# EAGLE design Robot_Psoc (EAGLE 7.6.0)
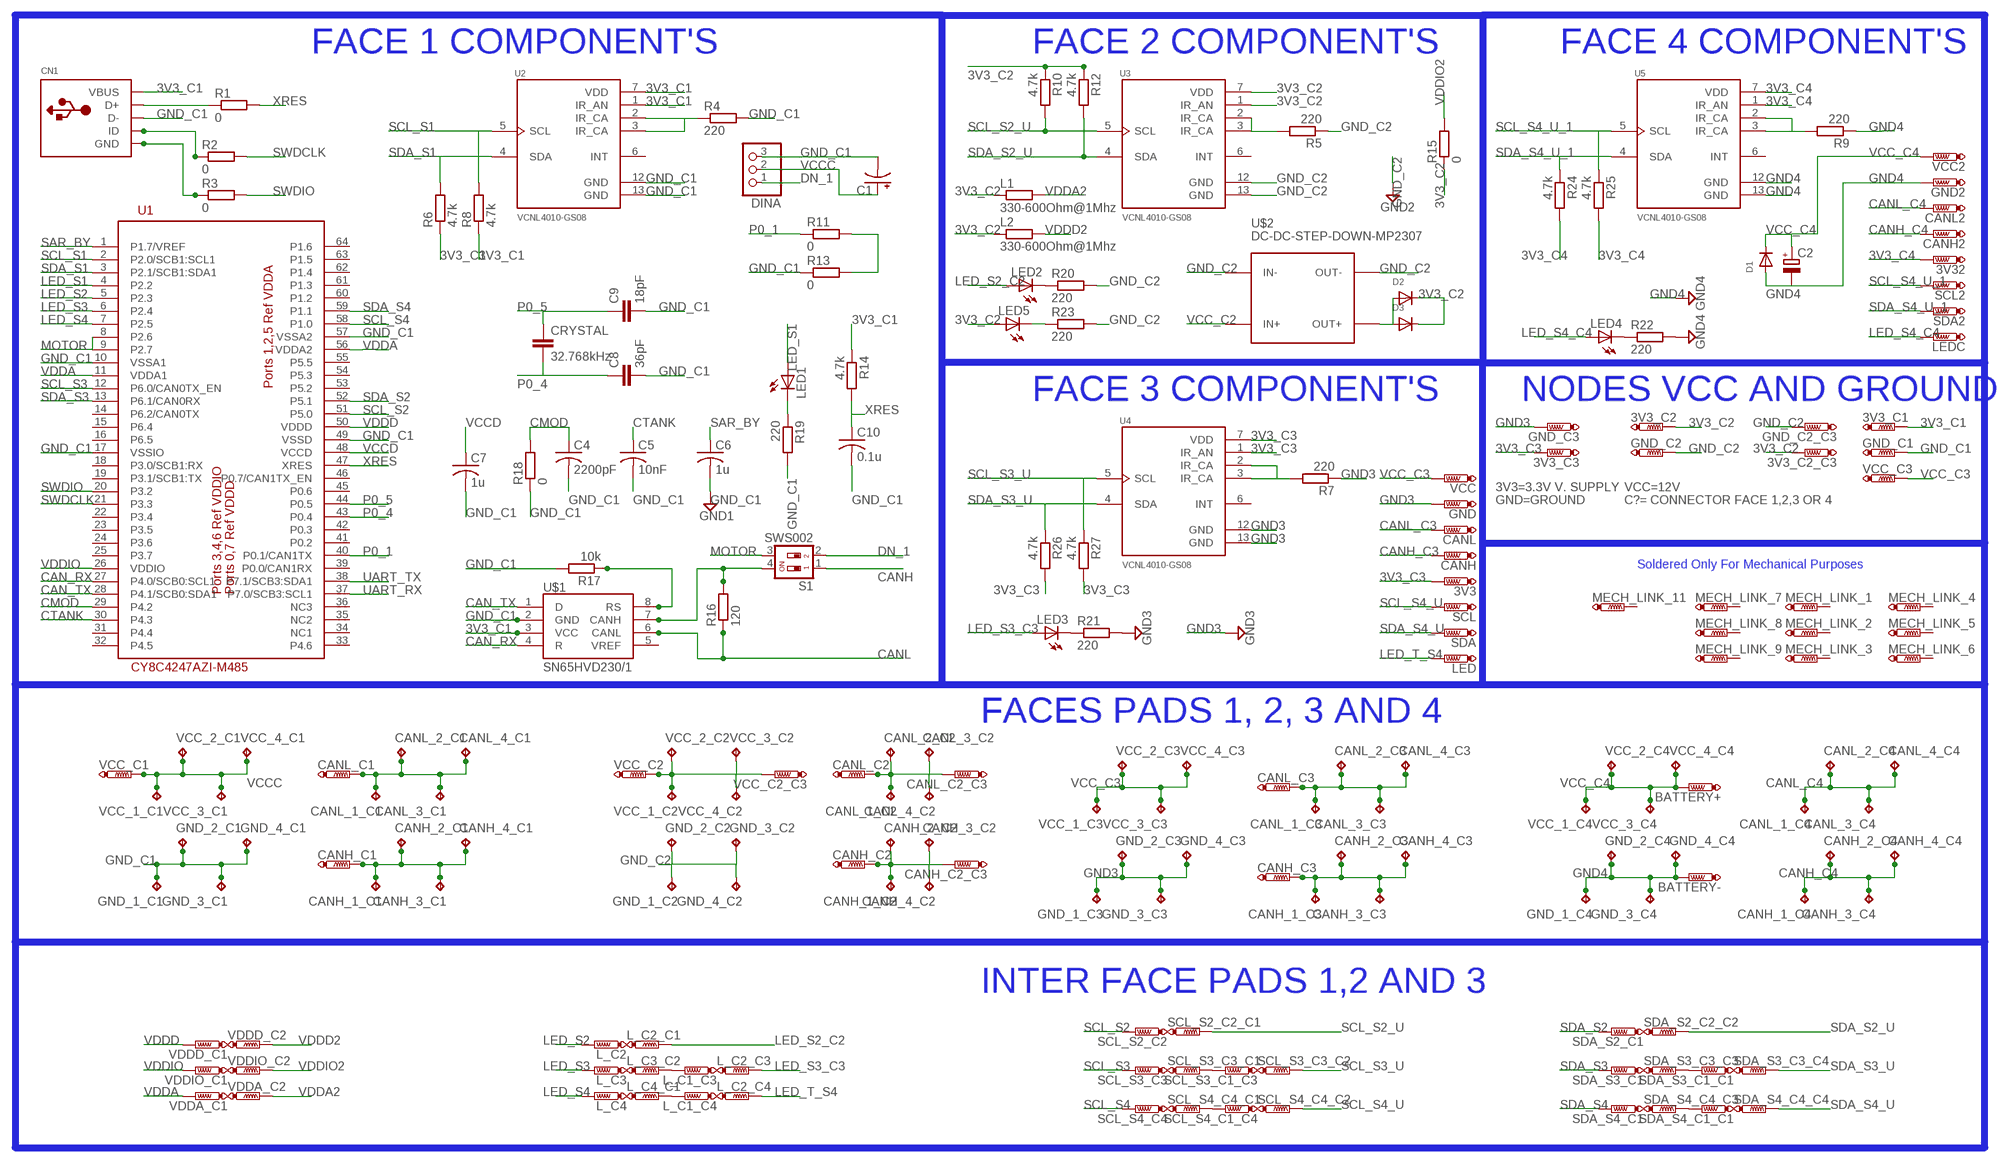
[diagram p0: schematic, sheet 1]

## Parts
3V3  PTR1TP11R  [TP11R]
3V3_C1  PTR1TP11R  [TP11R]
3V3_C2  PTR1TP11R  [TP11R]
3V3_C2_C3  PTR1TP11R  [TP11R]
3V3_C3  PTR1TP11R  [TP11R]
3V32  PTR1TP11R  [TP11R]
BATTERY+  PTR1TP11R  [TP11R]
BATTERY-  PTR1TP11R  [TP11R]
C1  CPOL-USUD-5X5,8  [UD-5X5,8_NICHICON]
C2  CPOL-EUUD-8X10  [UD-8X10_NICHICON]
C4  2200pF  C-USC0805  [C0805]
C5  10nF  C-USC0805  [C0805]
C6  1u  C-USC0805  [C0805]
C7  1u  C-USC0805  [C0805]
C8  36pF  C-EUC0805  [C0805]
C9  18pF  C-EUC0805  [C0805]
C10  0.1u  C-USC0805  [C0805]
CANH  PTR1TP11R  [TP11R]
CANH2  PTR1TP11R  [TP11R]
CANH_1_C1  TPB2,54  [B2,54]
CANH_1_C2  TPB2,54  [B2,54]
CANH_1_C3  TPB2,54  [B2,54]
CANH_1_C4  TPB2,54  [B2,54]
CANH_2_C1  TPB2,54  [B2,54]
CANH_2_C2  TPB2,54  [B2,54]
CANH_2_C3  TPB2,54  [B2,54]
CANH_2_C4  TPB2,54  [B2,54]
CANH_3_C1  TPB2,54  [B2,54]
CANH_3_C2  TPB2,54  [B2,54]
CANH_3_C3  TPB2,54  [B2,54]
CANH_3_C4  TPB2,54  [B2,54]
CANH_4_C1  TPB2,54  [B2,54]
CANH_4_C2  TPB2,54  [B2,54]
CANH_4_C3  TPB2,54  [B2,54]
CANH_4_C4  TPB2,54  [B2,54]
CANH_C1  PTR1TP11R  [TP11R]
CANH_C2  PTR1TP11R  [TP11R]
CANH_C2_C3  PTR1TP11R  [TP11R]
CANH_C3  PTR1TP11R  [TP11R]
CANL  PTR1TP11R  [TP11R]
CANL2  PTR1TP11R  [TP11R]
CANL_1_C1  TPB2,54  [B2,54]
CANL_1_C2  TPB2,54  [B2,54]
CANL_1_C3  TPB2,54  [B2,54]
CANL_1_C4  TPB2,54  [B2,54]
CANL_2_C1  TPB2,54  [B2,54]
CANL_2_C2  TPB2,54  [B2,54]
CANL_2_C3  TPB2,54  [B2,54]
CANL_2_C4  TPB2,54  [B2,54]
CANL_3_C1  TPB2,54  [B2,54]
CANL_3_C2  TPB2,54  [B2,54]
CANL_3_C3  TPB2,54  [B2,54]
CANL_3_C4  TPB2,54  [B2,54]
CANL_4_C1  TPB2,54  [B2,54]
CANL_4_C2  TPB2,54  [B2,54]
CANL_4_C3  TPB2,54  [B2,54]
CANL_4_C4  TPB2,54  [B2,54]
CANL_C1  PTR1TP11R  [TP11R]
CANL_C2  PTR1TP11R  [TP11R]
CANL_C2_C3  PTR1TP11R  [TP11R]
CANL_C3  PTR1TP11R  [TP11R]
CN1  USBMINIB  [USB-MINIB]
CRYSTAL  32.768kHz  C-EUC0603  [C0603]
D1  DIODESMA  [SMADIODE]
D2  DIODESOD-123  [SOD-123]
D3  DIODESOD-123  [SOD-123]
DINA  PINHD-1X3  [1X03]
GND  PTR1TP11R  [TP11R]
GND2  PTR1TP11R  [TP11R]
GND_1_C1  TPB2,54  [B2,54]
GND_1_C2  TPB2,54  [B2,54]
GND_1_C3  TPB2,54  [B2,54]
GND_1_C4  TPB2,54  [B2,54]
GND_2_C1  TPB2,54  [B2,54]
GND_2_C2  TPB2,54  [B2,54]
GND_2_C3  TPB2,54  [B2,54]
GND_2_C4  TPB2,54  [B2,54]
GND_3_C1  TPB2,54  [B2,54]
GND_3_C2  TPB2,54  [B2,54]
GND_3_C3  TPB2,54  [B2,54]
GND_3_C4  TPB2,54  [B2,54]
GND_4_C1  TPB2,54  [B2,54]
GND_4_C2  TPB2,54  [B2,54]
GND_4_C3  TPB2,54  [B2,54]
GND_4_C4  TPB2,54  [B2,54]
GND_C1  PTR1TP11R  [TP11R]
GND_C2  PTR1TP11R  [TP11R]
GND_C2_C3  PTR1TP11R  [TP11R]
GND_C3  PTR1TP11R  [TP11R]
L1  330-600Ohm@1Mhz  R-EU_R0805  [R0805]
L2  330-600Ohm@1Mhz  R-EU_R0805  [R0805]
L_C1_C3  PTR1TP11R  [TP11R]
L_C1_C4  PTR1TP11R  [TP11R]
L_C2  PTR1TP11R  [TP11R]
L_C2_C1  PTR1TP11R  [TP11R]
L_C2_C3  PTR1TP11R  [TP11R]
L_C2_C4  PTR1TP11R  [TP11R]
L_C3  PTR1TP11R  [TP11R]
L_C3_C2  PTR1TP11R  [TP11R]
L_C4  PTR1TP11R  [TP11R]
L_C4_C1  PTR1TP11R  [TP11R]
LED  PTR1TP11R  [TP11R]
LED1  LEDCHIPLED_0805  [CHIPLED_0805]
LED2  LEDCHIPLED_0805  [CHIPLED_0805]
LED3  LEDCHIPLED_0805  [CHIPLED_0805]
LED4  LEDCHIPLED_0805  [CHIPLED_0805]
LED5  LEDCHIPLED_0805  [CHIPLED_0805]
LEDC  PTR1TP11R  [TP11R]
MECH_LINK_1  PTR1TP11R  [TP11R]
MECH_LINK_2  PTR1TP11R  [TP11R]
MECH_LINK_3  PTR1TP11R  [TP11R]
MECH_LINK_4  PTR1TP11R  [TP11R]
MECH_LINK_5  PTR1TP11R  [TP11R]
MECH_LINK_6  PTR1TP11R  [TP11R]
MECH_LINK_7  PTR1TP11R  [TP11R]
MECH_LINK_8  PTR1TP11R  [TP11R]
MECH_LINK_9  PTR1TP11R  [TP11R]
MECH_LINK_11  PTR1TP11R  [TP11R]
R1  0  R-EU_R0805  [R0805]
R2  0  R-EU_R0805  [R0805]
R3  0  R-EU_R0805  [R0805]
R4  220  R-EU_R0805  [R0805]
R5  220  R-EU_R0805  [R0805]
R6  4.7k  R-EU_R0805  [R0805]
R7  220  R-EU_R0805  [R0805]
R8  4.7k  R-EU_R0805  [R0805]
R9  220  R-EU_R0805  [R0805]
R10  4.7k  R-EU_R0805  [R0805]
R11  0  R-EU_R0805  [R0805]
R12  4.7k  R-EU_R0805  [R0805]
R13  0  R-EU_R0805  [R0805]
R14  4.7k  R-EU_R0805  [R0805]
R15  0  R-EU_R0805  [R0805]
R16  120  R-EU_R0805  [R0805]
R17  10k  R-EU_R0805  [R0805]
R18  0  R-EU_R0805  [R0805]
R19  220  R-EU_R0805  [R0805]
R20  220  R-EU_R0805  [R0805]
R21  220  R-EU_R0805  [R0805]
R22  220  R-EU_R0805  [R0805]
R23  220  R-EU_R0805  [R0805]
R24  4.7k  R-EU_R0805  [R0805]
R25  4.7k  R-EU_R0805  [R0805]
R26  4.7k  R-EU_R0805  [R0805]
R27  4.7k  R-EU_R0805  [R0805]
S1  SWS002  [SMS-002]
SCL  PTR1TP11R  [TP11R]
SCL2  PTR1TP11R  [TP11R]
SCL_S2_C2  PTR1TP11R  [TP11R]
SCL_S2_C2_C1  PTR1TP11R  [TP11R]
SCL_S3_C1_C3  PTR1TP11R  [TP11R]
SCL_S3_C3  PTR1TP11R  [TP11R]
SCL_S3_C3_C1  PTR1TP11R  [TP11R]
SCL_S3_C3_C2  PTR1TP11R  [TP11R]
SCL_S4_C1_C4  PTR1TP11R  [TP11R]
SCL_S4_C4  PTR1TP11R  [TP11R]
SCL_S4_C4_C1  PTR1TP11R  [TP11R]
SCL_S4_C4_C2  PTR1TP11R  [TP11R]
SDA  PTR1TP11R  [TP11R]
SDA2  PTR1TP11R  [TP11R]
SDA_S2_C1  PTR1TP11R  [TP11R]
SDA_S2_C2_C2  PTR1TP11R  [TP11R]
SDA_S3_C1  PTR1TP11R  [TP11R]
SDA_S3_C1_C1  PTR1TP11R  [TP11R]
SDA_S3_C3_C3  PTR1TP11R  [TP11R]
SDA_S3_C3_C4  PTR1TP11R  [TP11R]
SDA_S4_C1  PTR1TP11R  [TP11R]
SDA_S4_C1_C1  PTR1TP11R  [TP11R]
SDA_S4_C4_C3  PTR1TP11R  [TP11R]
SDA_S4_C4_C4  PTR1TP11R  [TP11R]
U1  CY8C4247AZI-M485  [TQFP64-10X10]
U2  VCNL4010-GS08  [XDCR_VCNL4010-GS08]
U3  VCNL4010-GS08  [XDCR_VCNL4010-GS08]
U4  VCNL4010-GS08  [XDCR_VCNL4010-GS08]
U5  VCNL4010-GS08  [XDCR_VCNL4010-GS08]
U$1  SN65HVD230/1  [SO8]
U$2  DC-DC-STEP-DOWN-MP2307  [DC-DC-STEP-DOWN-MP2307]
VCC  PTR1TP11R  [TP11R]
VCC2  PTR1TP11R  [TP11R]
VCC_1_C1  TPB2,54  [B2,54]
VCC_1_C2  TPB2,54  [B2,54]
VCC_1_C3  TPB2,54  [B2,54]
VCC_1_C4  TPB2,54  [B2,54]
VCC_2_C1  TPB2,54  [B2,54]
VCC_2_C2  TPB2,54  [B2,54]
VCC_2_C3  TPB2,54  [B2,54]
VCC_2_C4  TPB2,54  [B2,54]
VCC_3_C1  TPB2,54  [B2,54]
VCC_3_C2  TPB2,54  [B2,54]
VCC_3_C3  TPB2,54  [B2,54]
VCC_3_C4  TPB2,54  [B2,54]
VCC_4_C1  TPB2,54  [B2,54]
VCC_4_C2  TPB2,54  [B2,54]
VCC_4_C3  TPB2,54  [B2,54]
VCC_4_C4  TPB2,54  [B2,54]
VCC_C1  PTR1TP11R  [TP11R]
VCC_C2  PTR1TP11R  [TP11R]
VCC_C2_C3  PTR1TP11R  [TP11R]
VCC_C3  PTR1TP11R  [TP11R]
VDDA_C1  PTR1TP11R  [TP11R]
VDDA_C2  PTR1TP11R  [TP11R]
VDDD_C1  PTR1TP11R  [TP11R]
VDDD_C2  PTR1TP11R  [TP11R]
VDDIO_C1  PTR1TP11R  [TP11R]
VDDIO_C2  PTR1TP11R  [TP11R]

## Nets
3V3_C1: 3V3_C1.TP CN1.VBUS R6.1 R8.1 R14.1 U2.1(IR_AN) U2.7(VDD) U$1.3(VCC)
3V3_C2: 3V3_C2.TP 3V3_C2_C3.TP D2.C D3.C L1.1 L2.1 LED5.A R10.1 R12.1 R15.1 U3.1(IR_AN) U3.7(VDD)
3V3_C3: 3V3.TP 3V3_C3.TP R26.2 R27.2 U4.1(IR_AN) U4.7(VDD)
3V3_C4: 3V32.TP R24.2 R25.2 U5.1(IR_AN) U5.7(VDD)
CAN_RX: U1.27(P4.0/SCB0:SCL1) U$1.4(R)
CAN_TX: U1.28(P4.1/SCB0:SDA1) U$1.1(D)
CANH: CANH_1_C1.TP CANH_2_C1.TP CANH_3_C1.TP CANH_4_C1.TP CANH_C1.TP S1.1
CANH_C3: CANH.TP CANH_1_C3.TP CANH_2_C3.TP CANH_3_C3.TP CANH_4_C3.TP CANH_C3.TP
CANH_C4: CANH2.TP CANH_1_C4.TP CANH_2_C4.TP CANH_3_C4.TP CANH_4_C4.TP
CANL: CANL_1_C1.TP CANL_2_C1.TP CANL_3_C1.TP CANL_4_C1.TP CANL_C1.TP R16.1 U$1.6(CANL)
CANL_C3: CANL.TP CANL_1_C3.TP CANL_2_C3.TP CANL_3_C3.TP CANL_4_C3.TP CANL_C3.TP
CANL_C4: CANL2.TP CANL_1_C4.TP CANL_2_C4.TP CANL_3_C4.TP CANL_4_C4.TP
CMOD: C4.1 R18.2 U1.29(P4.2)
CTANK: C5.1 U1.30(P4.3)
DN_1: DINA.1 S1.2
GND3: GND.TP GND_1_C3.TP GND_2_C3.TP GND_3_C3.TP GND_4_C3.TP GND_C3.TP R7.1 R21.2 U4.12(GND) U4.13(GND)
GND4: BATTERY-.TP C2.- D1.A GND2.TP GND_1_C4.TP GND_2_C4.TP GND_3_C4.TP GND_4_C4.TP R9.1 R22.2 U5.12(GND) U5.13(GND)
GND_C1: C1.- C4.2 C5.2 C6.2 C7.2 C8.2 C9.2 C10.2 CN1.D- DINA.3 GND_1_C1.TP GND_2_C1.TP GND_3_C1.TP GND_4_C1.TP GND_C1.TP R4.2 R13.1 R17.2 R18.1 R19.2 U1.10(VSSA1) U1.17(VSSIO) U1.49(VSSD) U1.57(VSSA2) U2.12(GND) U2.13(GND) U$1.2(GND) ; supply symbol labelled GND1
GND_C2: GND_1_C2.TP GND_2_C2.TP GND_3_C2.TP GND_4_C2.TP GND_C2.TP GND_C2_C3.TP R5.1 R20.2 R23.2 U3.12(GND) U3.13(GND) U$2.IN- U$2.OUT- ; supply symbol labelled GND2
LED_S1: LED1.A U1.4(P2.2)
LED_S2: L_C2.TP U1.5(P2.3)
LED_S2_C2: L_C2_C1.TP LED2.A
LED_S3: L_C3.TP U1.6(P2.4)
LED_S3_C3: L_C2_C3.TP LED3.A
LED_S4: L_C4.TP U1.7(P2.5)
LED_S4_C4: LED4.A LEDC.TP
LED_T_S4: L_C2_C4.TP LED.TP
MOTOR: S1.3 U1.8(P2.6) U1.9(P2.7)
N$1: CN1.D+ R1.1
N$2: CN1.ID R2.1
N$3: CN1.GND R3.1
N$4: R11.2 R13.2
N$5: R16.2 S1.4 U$1.7(CANH)
N$7: CANH_1_C2.TP CANH_2_C2.TP CANH_3_C2.TP CANH_4_C2.TP CANH_C2.TP CANH_C2_C3.TP
N$8: R7.2 U4.2(IR_CA) U4.3(IR_CA)
N$9: R17.1 U$1.8(RS)
N$10: SDA_S3_C1_C1.TP SDA_S3_C3_C3.TP
N$14: LED1.C R19.1
N$15: LED2.C R20.1
N$16: LED3.C R21.1
N$17: LED4.C R22.1
N$18: LED5.C R23.1
N$20: L_C1_C4.TP L_C4_C1.TP
N$21: R4.1 U2.2(IR_CA) U2.3(IR_CA)
N$22: L_C1_C3.TP L_C3_C2.TP
N$24: D2.A D3.A U$2.OUT+
N$26: SCL_S3_C1_C3.TP SCL_S3_C3_C1.TP
N$27: SCL_S4_C1_C4.TP SCL_S4_C4_C1.TP
N$32: CANL_1_C2.TP CANL_2_C2.TP CANL_3_C2.TP CANL_4_C2.TP CANL_C2.TP CANL_C2_C3.TP
N$43: R5.2 U3.2(IR_CA) U3.3(IR_CA)
N$44: SDA_S4_C1_C1.TP SDA_S4_C4_C3.TP
N$46: R9.2 U5.2(IR_CA) U5.3(IR_CA)
P0_1: R11.1 U1.40(P0.1/CAN1TX)
P0_4: C8.1 CRYSTAL.2 U1.43(P0.4)
P0_5: C9.1 CRYSTAL.1 U1.44(P0.5)
SAR_BY: C6.1 U1.1(P1.7/VREF)
SCL_S1: R8.2 U1.2(P2.0/SCB1:SCL1) U2.5(SCL)
SCL_S2: SCL_S2_C2.TP U1.51(P5.0)
SCL_S2_U: R10.2 SCL_S2_C2_C1.TP U3.5(SCL)
SCL_S3: SCL_S3_C3.TP U1.12(P6.0/CAN0TX_EN)
SCL_S3_U: R27.1 SCL_S3_C3_C2.TP U4.5(SCL)
SCL_S4: SCL_S4_C4.TP U1.58(P1.0)
SCL_S4_U: SCL.TP SCL_S4_C4_C2.TP
SCL_S4_U_1: R25.1 SCL2.TP U5.5(SCL)
SDA_S1: R6.2 U1.3(P2.1/SCB1:SDA1) U2.4(SDA)
SDA_S2: SDA_S2_C1.TP U1.52(P5.1)
SDA_S2_U: R12.2 SDA_S2_C2_C2.TP U3.4(SDA)
SDA_S3: SDA_S3_C1.TP U1.13(P6.1/CAN0RX)
SDA_S3_U: R26.1 SDA_S3_C3_C4.TP U4.4(SDA)
SDA_S4: SDA_S4_C1.TP U1.59(P1.1)
SDA_S4_U: SDA.TP SDA_S4_C4_C4.TP
SDA_S4_U_1: R24.1 SDA2.TP U5.4(SDA)
SWDCLK: R2.2 U1.21(P3.3)
SWDIO: R3.2 U1.20(P3.2)
UART_RX: U1.37(P7.0/SCB3:SCL1)
UART_TX: U1.38(P7.1/SCB3:SDA1)
VCC_C2: U$2.IN+ VCC_1_C2.TP VCC_2_C2.TP VCC_3_C2.TP VCC_4_C2.TP VCC_C2.TP VCC_C2_C3.TP
VCC_C3: VCC.TP VCC_1_C3.TP VCC_2_C3.TP VCC_3_C3.TP VCC_4_C3.TP VCC_C3.TP
VCC_C4: BATTERY+.TP C2.+ D1.C VCC2.TP VCC_1_C4.TP VCC_2_C4.TP VCC_3_C4.TP VCC_4_C4.TP
VCCC: C1.+ DINA.2 VCC_1_C1.TP VCC_2_C1.TP VCC_3_C1.TP VCC_4_C1.TP VCC_C1.TP
VCCD: C7.1 U1.48(VCCD)
VDDA: U1.11(VDDA1) U1.56(VDDA2) VDDA_C1.TP
VDDA2: L1.2 VDDA_C2.TP
VDDD: U1.50(VDDD) VDDD_C1.TP
VDDD2: L2.2 VDDD_C2.TP
VDDIO: U1.26(VDDIO) VDDIO_C1.TP
VDDIO2: R15.2 VDDIO_C2.TP
XRES: C10.1 R1.2 R14.2 U1.47(XRES)
Unconnected: MECH_LINK_1.TP MECH_LINK_2.TP MECH_LINK_3.TP MECH_LINK_4.TP MECH_LINK_5.TP MECH_LINK_6.TP MECH_LINK_7.TP MECH_LINK_8.TP MECH_LINK_9.TP MECH_LINK_11.TP U1.14(P6.2/CAN0TX) U1.15(P6.4) U1.16(P6.5) U1.18(P3.0/SCB1:RX) U1.19(P3.1/SCB1:TX) U1.22(P3.4) U1.23(P3.5) U1.24(P3.6) U1.25(P3.7) U1.31(P4.4) U1.32(P4.5) U1.33(P4.6) U1.34(NC1) U1.35(NC2) U1.36(NC3) U1.39(P0.0/CAN1RX) U1.41(P0.2) U1.42(P0.3) U1.45(P0.6) U1.46(P0.7/CAN1TX_EN) U1.53(P5.2) U1.54(P5.3) U1.55(P5.5) U1.60(P1.2) U1.61(P1.3) U1.62(P1.4) U1.63(P1.5) U1.64(P1.6) U2.6(INT) U3.6(INT) U4.6(INT) U5.6(INT) U$1.5(VREF)

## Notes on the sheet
- FACE 1 COMPONENT'S | FACE 2 COMPONENT'S | FACE 4 COMPONENT'S
- FACE 3 COMPONENT'S | NODES VCC AND GROUND
- 3V3=3.3V V. SUPPLY | VCC=12V
- GND=GROUND | C?= CONNECTOR FACE 1,2,3 OR 4
- Soldered Only For Mechanical Purposes
- FACES PADS 1, 2, 3 AND 4
- INTER FACE PADS 1,2 AND 3

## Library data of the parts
3V3 3V3_C1 3V3_C2 3V3_C2_C3 3V3_C3 3V32 BATTERY+ BATTERY- CANH CANH2 CANH_C1 CANH_C2 CANH_C2_C3 CANH_C3 CANL CANL2 CANL_C1 CANL_C2 CANL_C2_C3 CANL_C3 GND GND2 GND_C1 GND_C2 GND_C2_C3 GND_C3 L_C1_C3 L_C1_C4 L_C2 L_C2_C1 L_C2_C3 L_C2_C4 L_C3 L_C3_C2 L_C4 L_C4_C1 LED LEDC MECH_LINK_1-MECH_LINK_9 MECH_LINK_11 SCL SCL2 SCL_S2_C2 SCL_S2_C2_C1 SCL_S3_C1_C3 SCL_S3_C3 SCL_S3_C3_C1 SCL_S3_C3_C2 SCL_S4_C1_C4 SCL_S4_C4 SCL_S4_C4_C1 SCL_S4_C4_C2 SDA SDA2 SDA_S2_C1 SDA_S2_C2_C2 SDA_S3_C1 SDA_S3_C1_C1 SDA_S3_C3_C3 SDA_S3_C3_C4 SDA_S4_C1 SDA_S4_C1_C1 SDA_S4_C4_C3 SDA_S4_C4_C4 VCC VCC2 VCC_C1 VCC_C2 VCC_C2_C3 VCC_C3 VDDA_C1 VDDA_C2 VDDD_C1 VDDD_C2 VDDIO_C1 VDDIO_C2 = testpad:PTR1: TEST PIN
C1 = rcl:CPOL-US: POLARIZED CAPACITOR, American symbol
C2 = rcl:CPOL-EU: POLARIZED CAPACITOR, European symbol
C4-C7 C10 = rcl:C-US: CAPACITOR, American symbol
C8 C9 CRYSTAL = rcl:C-EU: CAPACITOR, European symbol
CANH_1_C1-CANH_1_C4 CANH_2_C1-CANH_2_C4 CANH_3_C1-CANH_3_C4 CANH_4_C1-CANH_4_C4 CANL_1_C1-CANL_1_C4 CANL_2_C1-CANL_2_C4 CANL_3_C1-CANL_3_C4 CANL_4_C1-CANL_4_C4 GND_1_C1-GND_1_C4 GND_2_C1-GND_2_C4 GND_3_C1-GND_3_C4 GND_4_C1-GND_4_C4 VCC_1_C1-VCC_1_C4 VCC_2_C1-VCC_2_C4 VCC_3_C1-VCC_3_C4 VCC_4_C1-VCC_4_C4 = testpad:TP: Test pad
CN1 = adafruit:USB: USB Connectors USBMINIB - Surface Mount Female Mini-B USB Connector 4UConnector: 06564 By microbuilder.eu Thru-hole RA Female Mini-B USB Connector 4UConnector: 18732 By ladyada.net
D1-D3 = adafruit:DIODE: Diode
DINA = pinhead:PINHD-1X3: PIN HEADER
L1 L2 R1-R27 = rcl:R-EU_: RESISTOR, European symbol
LED1-LED5 = adafruit:LED: LED
S1 = smd-special:SWS002: SMD Dip Switch 2 pol.
U1 = CypressPSoC:CY8C4247AZI-M485
U2-U5 = VCNL4010-GS08:VCNL4010-GS08
U$1 = texas_instruments:SN65HVD230/1
U$2 = diy-modules:DC-DC-STEP-DOWN-MP2307: DC/DC Step-Down Regulator based on MP2307DN chip MP2307 datasheet available here: https://cdn-shop.adafruit.com/datasheets/MP2307_r1.9.pdf Click here to find device on ebay.com

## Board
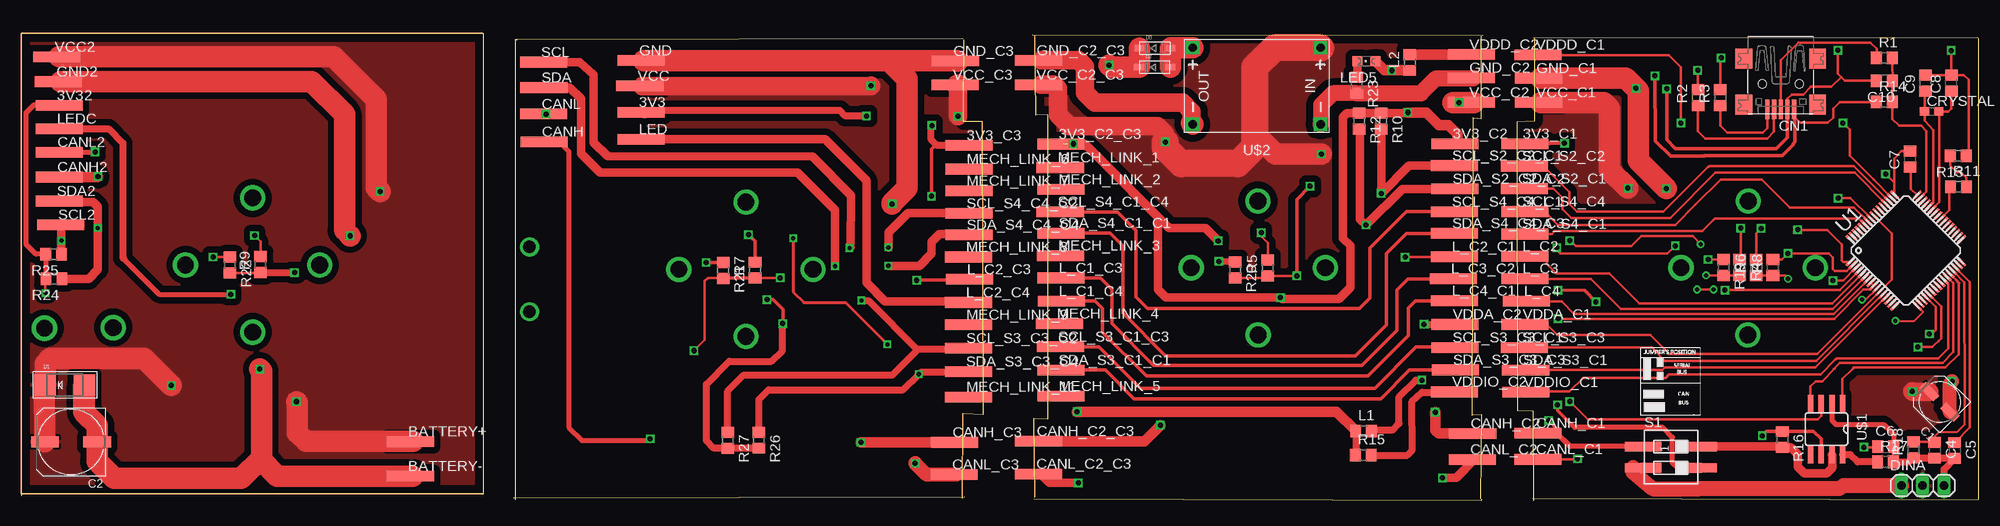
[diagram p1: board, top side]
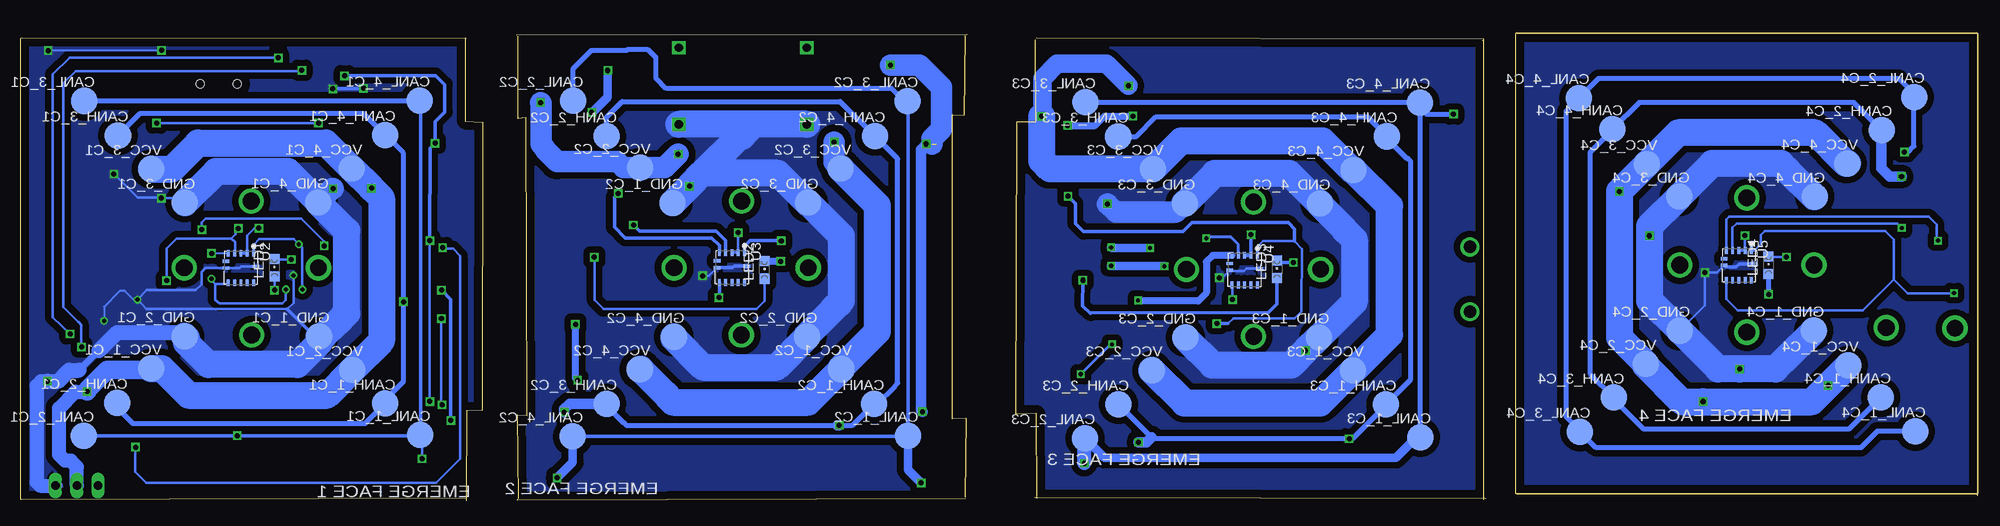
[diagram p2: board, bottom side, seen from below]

Size 233.48 x 55.82 mm. Coordinates in mm from the lower left corner, seen from the top.
Outline: 120.64,55.61 174.37,55.53
Outline: 112.44,55.01 112.4,45.25 114.65,45.24 114.75,10.31 112.3,10.39 112.28,0.29
Outline: 174.09,0.24 174.22,10.24 173.12,10.2 173.22,45.7 174.14,45.57 174.14,55.44
Outline: 120.84,55.49 120.94,46.04 122.4,46.1 122.4,9.76 120.75,9.84 120.86,0.38
Outline: 180.37,0 180.3,10.7 178.47,10.75 178.42,45.2 180.47,45.3 180.47,55.29
Outline: 0.01,0.55 0.01,55.55
Outline: 112.49,0.41 58.72,0.29
Outline: 112.33,55.19 58.97,55.08 58.97,0.08
Outline: 0,0.78 0,55.78
Outline: 233.37,55.26 180.34,55.2
Outline: 180.34,0.3 233.43,0.1
Outline: 233.48,0.17 233.48,55.17
Outline: 120.76,0.25 174.21,0.06 174.24,0.13
Outline: 59.12,54.99 59.01,54.99
Outline: 0.12,0.82 55.12,0.82 55.12,55.82 0.12,55.82
Outline: 55.01,0.82 0.01,0.82 0.01,55.82 55.01,55.82
Copper layers (1*16): Top 0.035mm / dielectric 1.5mm / Bottom 0.035mm
Design rules "default": minimum track width 10mil, minimum drill 24mil, track to track 8mil, track to pad 8mil, pad to pad 8mil, via to via 8mil, smd to smd 8mil, copper to edge 40mil, drill to drill 8mil, minimum pad ring 10mil, minimum via ring 8mil, stop-mask expansion 4mil, vias tented up to drill 0mil, thermal gap 10mil

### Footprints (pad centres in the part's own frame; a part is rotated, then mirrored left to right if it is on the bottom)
TP11R = smd 0.635 x 1.27: P$1 0.381,0; P$2 1.016,0; P$3 -0.254,0; P$4 -0.889,0; P$5 -1.524,0; P$6 1.613,0; P$7 2.21,0; P$8 -2.146,0; P$9 -2.769,0 | smd 1.1 x 1.1: TP 0,0
UD-5X5,8_NICHICON = smd 2.3 x 1: + 1.725,0; - -1.7,0
UD-8X10_NICHICON = smd 3.3 x 1.3: + 3.125,0; - -3.125,0
C0805 = smd 1.3 x 1.5: 1 -0.95,0; 2 0.95,0
B2,54 = smd 3.175 x 3.175 bottom: P$1 0,0 | smd 2.54 x 2.54 bottom: TP 0,0
USB-MINIB = smd 0.5 x 2.308: D+ 0,4.064; D- -0.8,4.064; GND 1.6,4.064; ID 0.8,4.064; VBUS -1.6,4.064 | smd 2 x 2.4: GND1 -4.4,-2; GND2 -4.4,3.5; GND3 4.4,3.5; GND4 4.4,-2 | hole 1: -2.2,1; 2.2,1
C0603 = smd 1.1 x 1: 1 -0.85,0; 2 0.85,0
SMADIODE = smd 2.54 x 2.54: A 2.349,0; C -2.349,0
SOD-123 = smd 1.2 x 0.7: A 1.85,0; C -1.85,0
1X03 = drill 1.016 long: 1 -2.54,0; 2 0,0; 3 2.54,0
R0805 = smd 1.3 x 1.5: 1 -0.95,0; 2 0.95,0
CHIPLED_0805 = smd 1.2 x 1.2: A 0,-1.05; C 0,1.05
SMS-002 = smd 1.092 x 2.007: 1 -1.27,-4.496; 2 1.27,-4.496; 3 1.27,4.496; 4 -1.27,4.496 | smd 1.143 x 2.54: P$1 -1.27,2.413; P$2 1.27,2.413; P$3 -1.27,-2.413; P$4 1.27,-2.413
TQFP64-10X10 = smd 1.2 x 0.3: 1 -5.7,3.75; 2 -5.7,3.25; 3 -5.7,2.75; 4 -5.7,2.25; 5 -5.7,1.75; 6 -5.7,1.25; 7 -5.7,0.75; 8 -5.7,0.25; 9 -5.7,-0.25; 10 -5.7,-0.75; 11 -5.7,-1.25; 12 -5.7,-1.75; 13 -5.7,-2.25; 14 -5.7,-2.75; 15 -5.7,-3.25; 16 -5.7,-3.75; 33 5.7,-3.75; 34 5.7,-3.25; 35 5.7,-2.75; 36 5.7,-2.25; 37 5.7,-1.75; 38 5.7,-1.25; 39 5.7,-0.75; 40 5.7,-0.25; 41 5.7,0.25; 42 5.7,0.75; 43 5.7,1.25; 44 5.7,1.75; 45 5.7,2.25; 46 5.7,2.75; 47 5.7,3.25; 48 5.7,3.75 | smd 0.3 x 1.2: 17 -3.75,-5.7; 18 -3.25,-5.7; 19 -2.75,-5.7; 20 -2.25,-5.7; 21 -1.75,-5.7; 22 -1.25,-5.7; 23 -0.75,-5.7; 24 -0.25,-5.7; 25 0.25,-5.7; 26 0.75,-5.7; 27 1.25,-5.7; 28 1.75,-5.7; 29 2.25,-5.7; 30 2.75,-5.7; 31 3.25,-5.7; 32 3.75,-5.7; 49 3.75,5.7; 50 3.25,5.7; 51 2.75,5.7; 52 2.25,5.7; 53 1.75,5.7; 54 1.25,5.7; 55 0.75,5.7; 56 0.25,5.7; 57 -0.25,5.7; 58 -0.75,5.7; 59 -1.25,5.7; 60 -1.75,5.7; 61 -2.25,5.7; 62 -2.75,5.7; 63 -3.25,5.7; 64 -3.75,5.7
XDCR_VCNL4010-GS08 = smd 0.805 x 0.35: 1 -1.772,1.5; 2 -1.772,0.75; 3 -1.772,0; 4 -1.772,-0.75; 5 -1.772,-1.5; 7 1.772,-1.5; 8 1.772,-0.75; 9 1.772,0; 10 1.772,0.75; 11 1.772,1.5 | smd 0.4 x 0.805: 6 -0.8,-1.772; 12 -0.175,1.772; 13 0,-1.772
SO8 = smd 0.66 x 2.032: 1 -1.905,-3.073; 2 -0.635,-3.073; 3 0.635,-3.073; 4 1.905,-3.073; 5 1.905,3.073; 6 0.635,3.073; 7 -0.635,3.073; 8 -1.905,3.073
DC-DC-STEP-DOWN-MP2307 = drill 1 pad 1.6 square: IN+ -7.62,-4.572; IN- -7.62,4.572; OUT+ 7.62,-4.572; OUT- 7.62,4.572

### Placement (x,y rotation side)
3V3  74.2,46.36 0 top
3V3_C1  179.65,42.6 0 top
3V3_C2  171.29,42.6 0 top
3V3_C2_C3  124.28,42.55 0 top
3V3_C3  113.3,42.39 0 top
3V32  4.77,47.17 0 top
BATTERY+  46.7,7.05 0 top
BATTERY-  46.68,2.91 0 top
C1  228.85,11.76 135 top
C2  5.91,7 180 top
C4  228.24,6.02 270 top
C5  230.63,5.97 270 top
C6  222.4,6.43 0 top
C7  225.32,40.77 90 top
C8  230.25,49.84 90 top
C9  227.17,49.84 90 top
C10  222.22,50.12 180 top
CANH  62.61,42.84 0 top
CANH2  4.79,38.61 0 top
CANH_1_C1  190.04,11.58 0 top
CANH_1_C2  131.73,11.53 0 top
CANH_1_C3  70.64,11.47 0 top
CANH_1_C4  11.62,12.33 0 top
CANH_2_C1  222,11.67 0 top
CANH_2_C2  163.62,43.48 0 top
CANH_2_C3  102.52,11.47 0 top
CANH_2_C4  11.48,44.25 0 top
CANH_3_C1  221.9,43.59 0 top
CANH_3_C2  163.62,11.55 0 top
CANH_3_C3  102.58,43.46 0 top
CANH_3_C4  43.44,12.3 0 top
CANH_4_C1  190.01,43.65 0 top
CANH_4_C2  131.6,43.52 0 top
CANH_4_C3  70.51,43.48 0 top
CANH_4_C4  43.61,44.33 0 top
CANH_C1  181.2,8.06 0 top
CANH_C2  173.4,8 0 top
CANH_C2_C3  121.64,7.09 0 top
CANH_C3  111.59,6.95 0 top
CANL  62.57,46.14 0 top
CANL2  4.8,41.59 0 top
CANL_1_C1  185.87,7.83 0 top
CANL_1_C2  127.66,7.73 0 top
CANL_1_C3  66.5,7.56 0 top
CANL_1_C4  7.48,8.27 0 top
CANL_2_C1  225.99,7.74 0 top
CANL_2_C2  167.63,47.73 0 top
CANL_2_C3  106.56,7.45 0 top
CANL_2_C4  7.6,48.19 0 top
CANL_3_C1  225.91,47.72 0 top
CANL_3_C2  127.68,47.68 0 top
CANL_3_C3  106.49,47.55 0 top
CANL_3_C4  47.48,8.21 0 top
CANL_4_C1  185.92,47.77 0 top
CANL_4_C2  167.65,7.66 0 top
CANL_4_C3  66.6,47.52 0 top
CANL_4_C4  47.6,48.06 0 top
CANL_C1  181.2,4.93 0 top
CANL_C2  173.35,4.91 0 top
CANL_C2_C3  121.59,3.18 0 top
CANL_C3  111.54,3.11 0 top
CN1  209.88,50.75 180 top
CRYSTAL  227.88,46.46 0 top
D1  5.17,13.8 0 top
D2  135.2,51.73 0 top
D3  135.23,54 0 top
DINA  226.82,1.78 0 top
GND  74.2,52.54 0 top
GND2  4.69,50.02 0 top
GND_1_C1  197.91,19.6 0 top
GND_1_C2  155.74,35.54 0 top
GND_1_C3  78.63,19.48 0 top
GND_1_C4  19.6,20.3 0 top
GND_2_C1  213.97,19.62 0 top
GND_2_C2  139.71,19.57 0 top
GND_2_C3  94.54,19.47 0 top
GND_2_C4  35.59,20.28 0 top
GND_3_C1  213.93,35.56 0 top
GND_3_C2  139.58,35.56 0 top
GND_3_C3  94.63,35.46 0 top
GND_3_C4  35.64,36.3 0 top
GND_4_C1  198.01,35.6 0 top
GND_4_C2  155.56,19.55 0 top
GND_4_C3  78.5,35.46 0 top
GND_4_C4  19.49,36.27 0 top
GND_C1  181.25,50.42 0 top
GND_C2  173.25,50.47 0 top
GND_C2_C3  121.61,52.56 0 top
GND_C3  111.69,52.47 0 top
L1  160.12,8.31 0 top
L2  165.63,52.3 90 top
L_C1_C3  124.3,26.57 0 top
L_C1_C4  124.33,23.8 0 top
L_C2  179.62,29.16 0 top
L_C2_C1  171.22,29.11 0 top
L_C2_C3  113.37,26.41 0 top
L_C2_C4  113.25,23.65 0 top
L_C3  179.65,26.5 0 top
L_C3_C2  171.12,26.5 0 top
L_C4  179.82,23.8 0 top
L_C4_C1  171.22,23.85 0 top
LED  74.2,43.14 0 top
LED1  203.22,27.79 0 bottom
LED2  144.78,27.54 0 bottom
LED3  83.63,27.61 0 bottom
LED4  25.01,28.11 0 bottom
LED5  160.45,52.45 90 top
LEDC  4.8,44.39 0 top
MECH_LINK_1  124.2,39.75 0 top
MECH_LINK_2  124.28,37.14 0 top
MECH_LINK_3  124.25,29.24 0 top
MECH_LINK_4  124.1,21.11 0 top
MECH_LINK_5  124.3,12.45 0 top
MECH_LINK_6  113.32,39.57 0 top
MECH_LINK_7  113.3,36.98 0 top
MECH_LINK_8  113.25,29.08 0 top
MECH_LINK_9  113.27,20.98 0 top
MECH_LINK_11  113.27,12.37 0 top
R1  222.22,52.84 0 top
R2  200,48.09 90 top
R3  202.66,48.11 90 top
R4  204.97,27.84 270 top
R5  148.69,27.77 90 top
R6  206.96,27.84 90 top
R7  87.52,27.51 90 top
R8  208.94,27.84 90 top
R9  28.51,28.19 90 top
R10  162.22,45.32 270 top
R11  231.09,37.47 0 top
R12  159.59,45.28 270 top
R13  231.06,41.15 180 top
R14  222.25,47.58 0 top
R15  160.07,5.43 0 top
R16  210.06,7.29 270 top
R17  222.37,4.63 0 top
R18  225.73,6.05 90 top
R19  203.04,27.84 270 top
R20  144.78,27.54 270 top
R21  83.71,27.48 270 top
R22  24.88,28.11 270 top
R23  159.31,49.57 270 top
R24  3.88,26.48 180 top
R25  3.82,29.41 180 top
R26  87.98,7.22 270 top
R27  84.26,7.21 270 top
S1  196.78,5.19 270 top
SCL  62.55,52.33 0 top
SCL2  4.94,32.93 0 top
SCL_S2_C2  179.57,39.93 0 top
SCL_S2_C2_C1  171.24,39.98 0 top
SCL_S3_C1_C3  124.25,18.37 0 top
SCL_S3_C3  179.6,18.27 0 top
SCL_S3_C3_C1  171.29,18.27 0 top
SCL_S3_C3_C2  113.27,18.19 0 top
SCL_S4_C1_C4  124.2,34.47 0 top
SCL_S4_C4  179.62,34.5 0 top
SCL_S4_C4_C1  171.22,34.47 0 top
SCL_S4_C4_C2  113.3,34.29 0 top
SDA  62.6,49.3 0 top
SDA2  4.79,35.75 0 top
SDA_S2_C1  179.57,37.24 0 top
SDA_S2_C2_C2  171.29,37.21 0 top
SDA_S3_C1  179.72,15.57 0 top
SDA_S3_C1_C1  124.28,15.57 0 top
SDA_S3_C3_C3  171.34,15.6 0 top
SDA_S3_C3_C4  113.25,15.39 0 top
SDA_S4_C1  179.61,31.83 0 top
SDA_S4_C1_C1  124.3,31.93 0 top
SDA_S4_C4_C3  171.24,31.91 0 top
SDA_S4_C4_C4  113.32,31.72 0 top
U1  224.81,29.85 45 top
U2  207.23,27.77 270 bottom
U3  148.66,27.82 270 bottom
U4  87.49,27.51 270 bottom
U5  28.54,28.09 270 bottom
U$1  215.34,8.54 180 top
U$2  147.37,49.49 180 top
VCC  74.05,49.5 0 top
VCC2  4.5,52.96 0 top
VCC_1_C1  217.94,15.77 0 top
VCC_1_C2  135.61,15.69 0 top
VCC_1_C3  74.56,15.54 0 top
VCC_1_C4  15.5,16.13 0 top
VCC_2_C1  193.94,15.6 0 top
VCC_2_C2  159.62,39.73 0 top
VCC_2_C3  98.56,15.55 0 top
VCC_2_C4  39.64,16.31 0 top
VCC_3_C1  217.94,39.59 0 top
VCC_3_C2  135.69,39.64 0 top
VCC_3_C3  98.43,39.59 0 top
VCC_3_C4  39.53,40.18 0 top
VCC_4_C1  194.01,39.64 0 top
VCC_4_C2  159.65,15.67 0 top
VCC_4_C3  74.5,39.47 0 top
VCC_4_C4  15.58,40.24 0 top
VCC_C1  181.25,47.53 0 top
VCC_C2  173.27,47.53 0 top
VCC_C2_C3  121.61,49.64 0 top
VCC_C3  111.66,49.62 0 top
VDDA_C1  179.63,21.03 0 top
VDDA_C2  171.29,21.03 0 top
VDDD_C1  181.2,53.22 0 top
VDDD_C2  173.27,53.24 0 top
VDDIO_C1  179.75,12.93 0 top
VDDIO_C2  171.22,12.98 0 top

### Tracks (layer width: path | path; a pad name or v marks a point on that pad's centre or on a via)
3V3_C1  (via drill 0.5, 0.6)
  Top 0.27: R8.1 210.36,26.89 v210.75,26.49 | v199.9,25.2 v201.87,25.2
  Top 0.305: 221.31,47.57 R14.1 216.94,47.58 216.14,46.79 216.14,45.73 215.51,45.1 212.18,45.1 211.54,45.74 | R6.1 R8.1 | v184.08,42.67 182.35,42.67 182.33,42.66 | U$1.3 214.7,10.12 214.28,9.69 186.88,9.68 v184.7,11.82 | v184.71,31.03 184.68,31.09 184.71,31.09 185.41,30.39 192.08,30.39 193.25,31.56 199.36,31.56 v200.34,30.59
  Top 0.406: 221.33,47.54 R14.1 | CN1.VBUS 211.54,46.62 211.54,45.74 211.54,42.77 211.41,42.63 211.41,42.5 210.08,41.17 200.79,41.17 200.74,41.13 196.78,41.13 194.91,42.9 v194.87,50.71
  Top 0.5: v184.08,42.67 182.33,42.66 179.48,42.61 3V3_C1.TP
  Bottom 0.27: v210.75,26.49 210.75,26.32 210.29,25.85 | 210.29,25.85 208.88,25.85 U2.7 | U2.1 205.74,30.51 205.04,31.21 200.96,31.21 | 200.96,31.21 199.93,30.19 199.93,25.49 v199.9,25.2 | v201.87,25.2 201.88,23.93 202.3,23.52 209.75,23.52 210.29,23.93 210.29,25.85 | 200.96,31.21 v200.34,30.59
  Bottom 0.305: 184.67,42.08 v184.08,42.67 | v184.7,11.82 184.69,30.49 v184.71,31.03
  Bottom 0.406: v184.71,31.03 184.67,42.08 | v184.08,42.67 184.08,45.22 182.93,46.37 182.93,49.66 184.02,50.75 v194.87,50.71
3V3_C2  (via drill 0.6)  (1 unrouted)
  Top 0.813: L1.1 159.17,5.34 R15.1
  Top 1.016: 135.58,33.84 135.58,25.18 136.52,24.24 v150.21,24.24 150.35,24.09 157.19,24.09 158.52,25.42 158.52,30.46 157.66,31.31 157.66,45.75 158.15,46.23 R12.1 162.19,46.23 R10.1 165.31,46.27 v165.39,46.34 | 135.58,33.84 133.17,36.25 | 135.58,33.84 136.9,32.52 141.25,32.52 v142.77,30.99 | 125.82,42.55 126.87,42.55 133.17,36.25 | 133.17,36.25 133.13,36.25 132.5,36.88 132.45,36.88 132.4,36.93
  Top 1.27: 3V3_C2.TP 171.29,43.75 170.22,44.82 169.11,44.82 167.63,46.3 165.45,46.3 v165.39,46.34 | L2.1 v163.48,51.35 162.6,51.35 LED5.A | L1.1 156.88,10.6 v125.93,10.6 | v125.49,42.59 125.82,42.55
  Top 2.54: D3.C 133.38,51.76 D2.C 130.04,51.73 v129.76,52.01
  Bottom 0.406: U3.7 150.16,24.28 v150.21,24.24 | U3.1 147.16,30.36 146.48,31.04 142.82,31.04 v142.77,30.99
  Bottom 1.016: v165.39,46.34 165.26,46.39 163.48,48.17 v163.48,51.35
  Bottom 1.27: v125.93,10.6 126.1,10.77 126.1,41.87 125.42,42.55 124.78,42.55 v125.49,42.59
  Bottom 2.54: 124.78,42.55 124.78,43.19 123.64,44.34 123.64,49.38 126.26,52.01 v129.76,52.01
3V3_C3  (via drill 0.6)
  Top 0.406: v88.94,23.98 89.67,23.98 90.84,22.82 90.84,21.15 v90.81,21.12 | v108.56,36.34 108.56,41.95 109.11,42.5
  Top 0.813: R26.2 R27.2 | R26.2 82.59,6.27 81.72,7.14 81.72,13.9 84.42,16.64 89.48,16.64 90.78,17.89 90.78,20.68 v90.81,21.12 | 87.75,6.04 R26.2 | 3V3_C3.TP 109.22,42.39 109.11,42.5 108.52,43.09 108.52,44.69 v108.61,44.78 | v100.82,45.92 98.27,45.92 97.63,46.56 74.4,46.56 3V3.TP
  Top 1.27: 74.34,46.23 3V3.TP
  Bottom 0.305: U4.1 85.99,30.28 85.31,30.96 81.55,30.96 80.67,30.05 80.71,23.02 80.71,22.58 81.56,21.74 88.86,21.74 89.47,21.12 | v88.94,23.98 88.94,25.68 U4.7
  Bottom 0.406: 81.55,30.96 81.55,32.43 82.3,33.18 93.76,33.18 94.85,32.09 106.7,32.09 107.7,33.1 107.7,35.47 v108.56,36.34 | v90.81,21.12 89.47,21.12
  Bottom 0.813: v108.61,44.78 105.33,44.78 104.24,45.87 100.86,45.87 v100.82,45.92
3V3_C4  (via drill 0.5)
  Top 0.305: v2.87,24.77 2.87,26.42 R24.2
  Top 0.61: 2.87,26.54 R25.2 1.73,29.41 0.55,30.59 0.55,46.3 1.5,47.25 4.7,47.25
  Top 1.016: 2.87,26.54 R24.2 | 4.7,47.25 3V32.TP
  Bottom 0.305: U5.1 26.66,29.86 25.91,30.61 25.91,31.69 25.44,32.17 11.06,32.17 10.04,31.15 10.04,26.41 | 10.04,26.41 8.36,24.73 2.9,24.73 v2.87,24.77 | U5.7 30.04,24.08 28.66,22.7 13.76,22.7 10.04,26.41
CAN_RX
  Top 0.27: 216.31,15.75 216.22,15.72 216.91,16.41 229.18,16.44 230.46,17.72 230.46,25.98 230.4,26.04
  Top 0.28: U$1.4 213.43,13.62 214.07,14.26 214.81,14.26 216.31,15.75
  Top 0.305: U1.27 229.73,26.66 229.78,26.66 230.4,26.04 | 213.51,11.69 U$1.4
CAN_TX
  Top 0.27: U$1.1 217.24,14.52 218.45,15.73 218.47,15.73 218.61,15.87 229.52,15.87 231.13,17.48 231.13,25.99 230.75,26.37
  Top 0.305: U1.28 230.75,26.37 231.16,25.96
CANH  (via drill 0.6)
  Top 0.406: S1.1 184.55,6.46 182.94,8.06 181.21,8.06 CANH_C1.TP | 183.13,8.08 183.13,8.63 v182.2,9.56 | v183.3,25.12 186.52,25.08 v187.83,23.72
  Top 0.61: S1.1 184.76,6.46 183.13,8.08
  Bottom 0.406: v182.2,9.56 182.2,24.02 v183.3,25.12
  Bottom 0.61: CANH_2_C1.TP 222,11.08 220.13,9.21 192.4,9.21 CANH_1_C1.TP 190.04,12.01 187.83,14.21 v187.83,23.72 187.83,41.47 CANH_4_C1.TP 190.05,43.65 192.59,46.19 219.3,46.19 CANH_3_C1.TP
CANH_C3  (via drill 0.6)
  Top 0.61: CANH.TP 64.15,42.84 65.3,41.68 65.3,8.75 66.87,7.17 74.82,7.17 v75.01,7.37
  Top 1.27: CANH_C3.TP v100.14,6.95
  Bottom 0.61: CANH_3_C3.TP 100.42,43.46 98.05,45.83 72.85,45.83 CANH_4_C3.TP 70.51,43.22 68.12,40.83 67.99,40.83 67.73,40.57 67.73,14.38 CANH_1_C3.TP 70.64,11.35 74.62,7.37 v75.01,7.37 98.42,7.37 98.61,7.56 CANH_2_C3.TP
  Bottom 1.27: v100.14,6.95 99.22,6.95 98.61,7.56
CANH_C4  (via drill 0.6)
  Top 1.27: CANH2.TP 9.04,38.61 v9.13,38.7
  Bottom 0.61: CANH_2_C4.TP 11.54,44.25 14.81,47.53 40.41,47.53 CANH_4_C4.TP 43.61,44.24 46.29,41.56 46.29,15.15 CANH_3_C4.TP 43.44,12.08 39.95,8.59 15.36,8.59 CANH_1_C4.TP
  Bottom 1.27: v9.13,38.7 10.55,38.7 11.53,39.68 11.53,44.2 CANH_2_C4.TP
CANL  (via drill 0.6)
  Top 0.305: CANL_C1.TP 185.59,4.93 v185.64,4.99
  Top 0.406: v207.68,7.74 208.17,8.24 R16.1 210.12,8.3 213.75,8.3 214.7,7.35 U$1.6
  Bottom 0.305: v185.64,4.99 185.64,6.9 186.12,7.39
  Bottom 0.406: CANL_2_C1.TP v207.68,7.74 186.48,7.74 | 186.48,7.74 185.81,8.41 | 185.81,8.41 185.81,7.89 CANL_1_C1.TP | 185.81,8.41 185.81,47.66 CANL_4_C1.TP | 185.69,6.96 186.12,7.39 186.48,7.74
  Bottom 0.61: CANL_3_C1.TP 185.97,47.72 CANL_4_C1.TP
CANL_C3  (via drill 0.6)
  Top 0.61: CANL.TP 63.94,46.14 64.02,46.23 62.66,46.23 CANL.TP
  Top 1.676: CANL_C3.TP 107.97,3.11 v106.62,4.45
  Bottom 0.61: CANL_3_C3.TP 66.63,47.55 CANL_4_C3.TP | CANL_4_C3.TP 66.6,7.65 CANL_1_C3.TP | 106.46,7.56 CANL_2_C3.TP | CANL_4_C3.TP 66.6,46.94 65.77,46.11 62.6,46.11 CANL.TP
  Bottom 1.016: CANL_1_C3.TP 67.01,7.56 69.43,5.13 104.24,5.13 CANL_2_C3.TP
  Bottom 1.676: v106.62,4.45 106.62,7.39 CANL_2_C3.TP
  other vias: 62.57,46.14
CANL_C4  (via drill 0.6)
  Top 0.61: CANL2.TP 8.74,41.59 v8.78,41.63
  Bottom 0.61: CANL_1_C4.TP 12.03,8.27 13.97,6.33 45.59,6.33 CANL_3_C4.TP 47.48,8.31 49.14,9.97 49.14,46.52 CANL_4_C4.TP 45.27,50.39 9.44,50.39 7.6,48.55 CANL_2_C4.TP 7.64,48.15 7.64,42.31 8.32,41.63 v8.78,41.63
CMOD
  Top 0.25: C4.1 228.24,7.67 228.79,8.21 230.94,8.21 231.85,9.12 231.85,11.45 231.83,11.47
  Top 0.305: U1.29 231.8,26.04 231.83,11.47 | 227.86,7 R18.2
  Top 0.813: 227.86,7 C4.1
CTANK
  Top 0.305: U1.30 232.46,26.09 232.46,8.73 C5.1
DN_1
  Top 1.778: DINA.1 217.38,1.78 216.82,1.41 200.16,1.41 199.99,1.42 194.58,1.42 192.29,3.34 S1.2
GND3  (via drill 0.6)
  Top 0.305: R7.1 90.48,26.56 v90.52,26.59 81.89,26.59 81.5,26.21 81.5,19.18 v80.22,17.9
  Top 0.406: R21.2 83.73,26.56 R7.1
  Top 2.54: GND.TP 103.51,52.54 | 103.51,52.54 111.62,52.54 GND_C3.TP | v103.87,35.42 103.87,35.52 105.65,37.29 105.65,50.4 103.51,52.54
  Bottom 0.305: U4.12 87.27,27.68 87.57,27.39 89.14,27.39 U4.13 90.18,26.59 v90.52,26.59 | v80.22,17.9 77.28,20.84
  Bottom 2.54: 82.17,39.06 91.03,39.06 95.67,34.42 102.87,34.42 v103.87,35.42
  Bottom 3.2: GND_2_C3.TP 94.54,19.36 91.36,16.18 81.94,16.18 v80.22,17.9 GND_1_C3.TP 77.28,20.84 74.42,23.69 74.42,31.17 75.54,32.28 75.54,32.35 78.5,35.31 GND_4_C3.TP 78.57,35.46 82.17,39.06 91.04,39.06 GND_3_C3.TP
  pour Bottom (isolate 0.762): 58.82,0.09 112.34,-0.08 112,10.16 114.61,10.39 114.71,45.21 112.58,45.25 112.23,55.15 58.69,55.35
GND4  (via drill 0.6)
  Top 0.305: R22.2 28.43,27.16 R9.1
  Top 0.813: R9.1 32.57,27.24 v32.58,27.22
  Top 2.54: C2.- 9.04,8.97 7.43,10.58 7.43,13.71 D1.A 7.52,10.46 9.02,8.96 9.02,4.68 11.04,2.66 26.24,2.66 28.65,5.07 | GND2.TP 34.62,50.02 38.54,46.11 38.54,32.27 v39.2,31.61 | BATTERY-.TP 30.53,2.91 28.65,4.8 28.65,5.07 | 28.65,5.07 28.65,15.48 v28.43,15.7
  Bottom 0.305: U5.13 31.17,27.22 v32.58,27.22 32.58,23.29 GND_2_C4.TP
  Bottom 0.406: U5.12 28.51,28.26 28.87,27.9 30.12,27.9 U5.13
  Bottom 3.2: GND_1_C4.TP 19.6,20.27 23.03,16.83 24.17,15.7 v28.43,15.7 31.01,15.7 GND_2_C4.TP 39.2,23.89 v39.2,31.61 39.2,32.75 GND_3_C4.TP | GND_3_C4.TP | GND_4_C4.TP 19.55,36.27 22.75,39.47 22.75,39.48 23.51,40.23 31.71,40.23 GND_3_C4.TP
  pour Bottom (isolate 0.762): -0.02,0.73 54.92,0.58 55.05,55.28 -0.02,55.34 -0.01,7.82
GND_C1  (via drill 0.5, 0.6)
  Top 0.25: U1.10 220.04,24.02 219.59,24.02 v219.57,24 | v223.56,21.45 225.82,21.45 226.86,22.49 226.86,22.5 U1.17
  Top 0.27: R4.2 201.29,26.89 v200.96,26.89
  Top 0.28: U1.49 223.43,40.85 224.27,41.69 225.29,41.69 C7.2
  Top 0.305: 225.73,5.02 R18.1 226.49,5.07 | R17.2 223.25,6.15 C6.2 | U1.17 | U1.10 | 228.42,5.02 C4.2 | R19.2 R4.2 | C9.2 C8.2 | C8.2 231.74,50.79 232.28,50.25 232.28,41.42 R13.1 | CN1.D- 210.68,47.97 211.18,48.47 212.55,48.47 213.46,49.39 215.91,49.39 217.09,50.57 | v216.71,53.75 216.67,53.68 216.67,50.99 217.09,50.57 | v230.22,53.72 230.22,50.81 C8.2 | C10.2 217.54,50.12 217.09,50.57 | U1.57 218.2,36.1 v216.73,36.1 | U1.49 223.43,37.95 v222.4,38.98
  Top 0.406: CN1.D- 210.68,43.36 209.36,42.04 197.33,42.04 196.28,43.09 v196.28,49.16 | v192.61,49.23 192.61,48.41 192.91,48.11
  Top 0.61: U$1.2 215.97,9.56 216.44,9.09 222.17,9.09 223.37,7.88 223.37,6.45 C6.2
  Top 0.813: 228.42,5.02 C5.2 229.36,3.75 DINA.3 | C4.2 226.49,5.07 | R17.2 225.08,4.6 R18.1
  Top 1.676: C1.- 230.05,13.97 v230.33,14.25
  Top 2.54: GND_C1.TP 191.41,50.42 v192.61,49.23 192.91,48.93 192.91,48.11 192.91,40.58 v196.23,37.25
  Bottom 0.25: v219.57,24 220.06,24 221.1,25.04 221.67,25.04 223.56,23.14 v223.56,21.45
  Bottom 0.27: U2.13 211.48,27.77 211.93,27.32 211.93,25.79 212.6,25.11 218.45,25.11 v219.57,24 218.51,22.85 201.69,22.85 200.96,23.58 v200.96,26.89
  Bottom 0.305: U2.13 207.39,27.77 207.21,27.94 U2.12 | v216.71,53.75 v230.22,53.72 | GND_3_C1.TP 214.47,36.1 v216.73,36.1 216.8,36.17 219.57,36.17 222.38,38.98 v222.4,38.98
  Bottom 0.406: GND_1_C1.TP 198.43,19.6 201.69,22.85 | v196.28,49.16 192.68,49.16 v192.61,49.23
  Bottom 0.813: 228.43,14.82 228.43,14.88 | 226.57,15.55 224.19,17.92 224.17,17.92
  Bottom 1.676: v230.33,14.25 231.07,14.25 231.62,13.69 231.62,2.19 231.2,1.77 229.37,1.77 DINA.3 | 214.42,20.07 GND_2_C1.TP
  Bottom 1.778: v230.33,14.25 229,14.25 228.43,14.82 | 228.43,14.88 227.77,15.55 226.57,15.55 | 224.17,17.92 222.01,20.07 214.42,20.07
  Bottom 2.54: v196.23,37.25 196.36,37.25 GND_4_C1.TP
  Bottom 3.2: GND_2_C1.TP 213.76,19.41 213.76,18.87 211.13,16.24 200.47,16.24 197.91,18.8 GND_1_C1.TP 197.39,19.6 195.76,21.23 194.62,22.38 194.62,32.21 GND_4_C1.TP 198.01,35.69 201.62,39.3 210.19,39.3 GND_3_C1.TP
  pour Bottom (isolate 0.762): 180.33,54.99 180.43,44.88 178.35,45 178.53,10.45 180.2,10.47 180.23,0.21 233.05,0.03 233.05,55.02
GND_C2  (via drill 0.6)
  Top 0.305: R20.2 148.46,26.59 R5.1 v152.14,26.82
  Top 0.406: v152.14,26.82 152.14,35.94 v153.74,37.54
  Top 1.93: GND_C2.TP 173.2,50.42 168.76,50.42 166.96,48.62 R23.2 156.44,48.62 155.04,47.22 155.04,44.96 U$2.IN-
  Top 2.184: GND_C2_C3.TP 126.12,52.56 126.86,51.81 126.86,48.7 128.08,47.48 138.56,47.48 139.58,46.46 139.58,45.08
  Top 2.54: 139.58,45.08 U$2.OUT-
  Bottom 0.305: v152.14,26.82 151.43,26.82 U3.13
  Bottom 0.406: U3.12 146.92,28.02 148.36,28.02 148.56,27.82 U3.13
  Bottom 3.2: GND_4_C2.TP 155.56,19.4 152.07,15.91 143.36,15.91 GND_2_C2.TP 139.71,19.7 136.6,22.81 136.6,22.87 135.61,23.86 135.61,31.6 GND_3_C2.TP 139.69,35.56 143.21,39.08 152.19,39.08 | 152.19,39.08 v153.74,37.54 GND_1_C2.TP | U$2.IN- U$2.OUT- 146.01,44.92 147.43,43.5 147.78,43.5 152.19,39.08
  pour Bottom (isolate 0.813): 120.92,0.57 174.17,0.18 174.25,10.38 173.15,10.36 173.24,45.84 174.11,45.73 174.02,55.49 120.77,55.41 120.95,46.13 122.29,45.81 122.18,9.93 120.82,9.89
LED_S1  (via drill 0.6)
  Top 0.305: v203.22,25.12 216.91,25.12 U1.4
  Bottom 0.305: LED1.A v203.22,25.12
LED_S2
  Top 0.305: U1.5 216.04,23.55 193.04,23.55 189.46,27.13 183.1,27.13 181.99,28.25 181.99,28.6 181.44,29.15 | 181.66,29.15 181.44,29.15 | 181.44,29.15 179.63,29.15 L_C2.TP
LED_S2_C2  (via drill 0.6)
  Top 0.305: v165.1,29.06 171.17,29.06 L_C2_C1.TP
  Bottom 0.305: LED2.A 144.78,23.83 145.72,22.89 163.98,22.89 165.02,23.93 165.02,28.99 v165.1,29.06
LED_S3
  Top 0.305: U1.6 216.08,22.89 190.79,22.89 187.24,26.44 181.23,26.44 181.2,26.47 179.67,26.47 L_C3.TP
LED_S3_C3  (via drill 0.6)
  Top 0.406: v106.8,26.31 113.27,26.31 L_C2_C3.TP
  Bottom 0.406: LED3.A 83.63,23.46 84.64,22.45 105.9,22.41 105.88,22.36 106.82,23.26 v106.8,26.31
LED_S4
  Top 0.305: U1.7 216.19,22.29 185.2,22.29 183.74,23.74 179.88,23.74 L_C4.TP
LED_S4_C4  (via drill 0.6)
  Top 0.61: 12.08,29 12.23,28.85 16.45,24.62 v24.98,24.62
  Top 0.813: LEDC.TP 10.39,44.39 12.08,42.69 12.08,28.99 12.23,28.85
  Bottom 0.61: v24.98,24.62 24.98,27.04 LED4.A
LED_T_S4
  Top 1.016: LED.TP 95.84,43.14 100.79,38.19 100.79,26.05 103.05,23.78 113.11,23.78 L_C2_C4.TP
MOTOR  (via drill 0.6)
  Top 0.305: U1.8 U1.9 220.51,25.2 219.73,25.2 216.24,21.7 183.34,21.7 v183.32,21.72
  Top 0.406: S1.3 199.31,3.92 | 185.34,8.68 185.05,8.97 183.28,10.73 v183.25,11.43
  Top 0.61: 199.31,3.92 197.52,3.92 196.96,4.47 196.96,7.58 195.82,8.72 185.29,8.72 185.05,8.97
  Bottom 0.305: v183.32,21.72 183.32,11.84 v183.25,11.43
N$1
  Top 0.305: CN1.D+ 209.88,52.57 211.98,54.68 220.59,54.68 221.32,53.95 221.32,52.88 R1.1
N$2
  Top 0.305: R2.1 200,44.1 200.86,43.23 208.25,43.23 209.04,44.02 209.04,46.65 CN1.ID
N$3
  Top 0.305: CN1.GND 208.28,44.48 207.72,43.92 203.53,43.92 202.69,44.76 202.69,47.14 R3.1
N$4
  Top 0.305: R13.2 230.11,39.97 230.86,39.22 231.37,39.22 232,38.59 232,37.5 R11.2
N$5
  Top 0.406: 216.02,5.52 U$1.7
  Top 1: S1.4 209.94,6.46 R16.2 211.08,6.34 211.89,5.52 211.89,4.05 212.7,3.24 215.34,3.24 216.01,3.9 216.01,5.43 U$1.7
N$6  (via drill 2)
  other vias: 206,35.77
N$7  (via drill 0.6)
  Top 1.27: CANH_C2.TP 169.07,8 168.67,8.41 v168.67,10.56 | CANH_C2_C3.TP 133.94,7.09 v135.86,9.01
  Bottom 0.61: CANH_2_C2.TP 163.62,45.78 161.74,47.65 135.74,47.65 CANH_4_C2.TP 128.89,40.8 128.89,14.02 129.16,13.75 129.16,13.71 131.33,11.53 CANH_1_C2.TP 134.25,9.01 v135.86,9.01 | CANH_3_C2.TP 163.62,11.29 161.65,9.33 161.6,9.33 161.28,9.01 136.04,9.01
  Bottom 1.27: v168.67,10.56 168.67,10.92 168.03,11.56 CANH_3_C2.TP | v135.86,9.01 136.04,9.01
N$8  (via drill 0.6)
  Top 0.406: R7.2 87.52,30.96 v86.73,31.75
  Bottom 0.406: U4.3 U4.2 v86.73,31.75
N$9
  Top 0.813: R17.1 219.05,4.63 218.18,5.46 U$1.8
N$10
  Top 0.406: SDA_S3_C1_C1.TP 129.31,15.57 132.71,12.17 162.18,12.17 165.58,15.57 171.32,15.57 SDA_S3_C3_C3.TP
N$11  (via drill 0.6)
  other vias: 212.06,49.74
N$12  (via drill 0.6)
  other vias: 207.67,49.74
N$13  (via drill 1.5)
  other vias: 60.62,30.28
N$14  (via drill 0.6)
  Top 0.305: R19.1 201.35,28.79 v201.21,28.78
  Bottom 0.305: v201.21,28.78 203.16,28.78 LED1.C
N$15  (via drill 0.6)
  Top 0.813: v142.85,28.55 144.69,28.58 R20.1
  Bottom 0.813: LED2.C 142.98,28.59 v142.85,28.55
N$16  (via drill 0.6)
  Top 0.406: R21.1 81.71,28.43 v81.67,28.42
  Bottom 0.406: v81.67,28.42 83.39,28.42 LED3.C
N$17  (via drill 0.6)
  Top 0.305: R22.1 22.86,29.06 v22.85,29.08
  Bottom 0.305: v22.85,29.08 24.92,29.08 LED4.C
N$18
  Top 1.016: LED5.C 159.4,50.62 R23.1
N$19  (via drill 1.5)
  other vias: 60.62,22.55
N$20
  Top 0.406: L_C1_C4.TP 128.09,23.8 128.98,22.91 128.98,20.1 134.21,14.86 160.6,14.86 165.45,19.71 165.45,22.99 166.29,23.83 171.19,23.83 L_C4_C1.TP
N$21  (via drill 0.6)
  Top 0.305: v205.1,32.52 205.1,28.84 R4.1
  Bottom 0.305: U2.2 206.49,31.64 205.63,32.49 205.13,32.49 v205.1,32.52
  Bottom 0.406: U2.2 U2.3
N$22
  Top 0.406: L_C1_C3.TP 128.72,26.57 130.09,25.2 130.09,21.14 135.07,16.16 159.94,16.16 164.08,20.3 164.08,25.15 165.38,26.45 171.06,26.45 L_C3_C2.TP
N$23  (via drill 2 pad 2.18)
  other vias: 213.99,27.79
N$24
  Top 2.54: U$2.OUT+ 137.14,54.06 D3.A 137.05,53.97 D2.A
N$25  (via drill 2 pad 2.18)
  other vias: 197.99,27.79
N$26
  Top 0.406: SCL_S3_C1_C3.TP 128.55,18.37 133.5,13.42 161.46,13.42 166.37,18.32 171.24,18.32 SCL_S3_C3_C1.TP
N$27
  Top 0.406: SCL_S4_C1_C4.TP 130.73,34.47 132.97,32.24 132.97,24.31 134.34,22.94 159.63,22.94 160.85,24.16 160.85,30.13 165.25,34.52 171.17,34.52 SCL_S4_C4_C1.TP
N$28  (via drill 2 pad 2.18)
  other vias: 205.96,19.79
N$29  (via drill 2)
  other vias: 2.75,20.58
N$30  (via drill 2 pad 2.18)
  other vias: 139.54,27.79
N$31  (via drill 2 pad 2.18)
  other vias: 147.49,35.77
N$32  (via drill 0.6)
  Top 1.016: CANL_C2.TP 171.16,2.72 v169.52,2.72 | CANL_C2_C3.TP 122.65,2.11 v126.1,2.11
  Bottom 0.406: CANL_4_C2.TP 127.73,7.66 CANL_1_C2.TP 127.66,47.66 CANL_3_C2.TP | 167.59,47.68 CANL_2_C2.TP
  Bottom 0.61: 167.59,47.68 167.6,47.7 167.6,51.57 165.41,53.76 161.2,53.76 161.15,53.81 158.64,53.81 157.73,52.9 157.73,50.44 156.5,49.2 129.62,49.2 128.1,47.68 CANL_3_C2.TP
  Bottom 1.016: v169.52,2.72 167.65,4.58 CANL_4_C2.TP | v126.1,2.11 127.66,3.68 CANL_1_C2.TP
N$33  (via drill 2 pad 2.18)
  other vias: 155.55,27.79
N$34  (via drill 2 pad 2.18)
  other vias: 147.54,19.79
N$35  (via drill 2)
  other vias: 78.42,27.61
N$36  (via drill 2)
  other vias: 86.42,35.63
N$37  (via drill 2)
  other vias: 94.43,27.61
N$38  (via drill 2)
  other vias: 86.42,19.61
N$39  (via drill 2)
  other vias: 19.57,28.14
N$40  (via drill 2)
  other vias: 27.57,36.14
N$41  (via drill 2)
  other vias: 35.57,28.14
N$42  (via drill 2)
  other vias: 27.57,20.11
N$43  (via drill 0.6)
  Top 0.305: R5.2 148.69,30.76 147.95,31.5 v147.92,31.98
  Bottom 0.305: v147.92,31.98 147.95,29.65 U3.2 U3.3
N$44
  Top 0.406: SDA_S4_C1_C1.TP 129.84,31.93 131.39,30.38 131.39,22.38 136.5,17.28 159.15,17.28 162.84,20.96 162.84,29.49 165.25,31.91 SDA_S4_C4_C3.TP
N$45  (via drill 2)
  other vias: 10.95,20.65
N$46  (via drill 0.6)
  Top 0.305: R9.2 28.51,30.93 v27.8,31.64
  Bottom 0.305: U5.3 U5.2 v27.8,31.64
P0_1
  Top 0.305: U1.40 229.99,34.67 229.99,37.33 R11.1
P0_4
  Top 0.305: U1.43 227.97,34.76 228.8,35.64 228.8,46.32 CRYSTAL.2 229.89,46.46 230.25,46.82 C8.1
P0_5
  Top 0.305: U1.44 227.62,35.12 228.06,35.56 228.06,44.23 227.05,45.34 227.05,46.45 CRYSTAL.1 227.04,48.75 C9.1
SAR_BY  (via drill 0.6)
  Top 0.305: U1.1 217.35,28.47 217.15,28.67 217.15,30.59 215.45,32.29 211.95,32.29 v211.9,32.34 | v219.8,6.38 221.4,6.38 C6.1 | v197.3,30.41 196.37,29.48 183.6,29.48 183.17,29.91 v183.17,30.19
  Bottom 0.305: v211.9,32.34 211.9,33.17 211.41,33.65 200.37,33.65 200.34,33.69 200.06,33.69 197.3,30.93 v197.3,30.41 | 219.7,6.3 v219.8,6.38 219.83,6.36 219.83,3.43 218.51,2.11 183.95,2.11 181.05,5.01 181.05,29.22 181.93,30.1 183.08,30.1 v183.17,30.19
SCL_S1  (via drill 0.6)
  Top 0.305: U1.2 218.48,28.09 217.78,27.39 216.35,27.39 216.07,27.66 216.07,29.04 215.59,29.52 v210.74,29.52 210.01,28.79 R8.2
  Bottom 0.305: v210.74,29.52 U2.5
SCL_S2
  Top 0.305: U1.51 218.59,39.96 201.36,39.96 201.24,39.84 201.21,39.84 195.85,34.48 185.56,34.48 184.65,35.39 184.65,36.84 181.94,39.55 181.94,39.93 SCL_S2_C2.TP
SCL_S2_U  (via drill 0.6)
  Top 1.016: SCL_S2_C2_C1.TP 165.54,39.98 v162.22,36.66 R10.2
  Bottom 0.406: U3.5 150.16,30.45 151.08,31.37 161.39,31.37 162.66,32.64 162.66,36.22 v162.22,36.66
SCL_S3
  Top 0.305: SCL_S3_C3.TP 194.48,18.27 196.06,16.69 214.13,16.69 U1.12
SCL_S3_U  (via drill 0.5)
  Top 0.813: R27.1 84.25,13.09 86.16,15 103.91,15 106.93,18.01 | 106.93,18.01 107.02,18.1 113.19,18.1 SCL_S3_C3_C2.TP | v100.21,23.89 101.05,23.89 106.93,18.01
  Bottom 0.813: U4.5 91.3,29.28 92.06,28.52 92.06,24.8 93.03,23.83 100.15,23.83 v100.21,23.89
SCL_S4
  Top 0.305: SCL_S4_C4.TP 181.71,34.5 183.28,32.92 197.3,32.92 199.71,35.33
  Top 0.32: 198.87,34.5 199.71,35.33 202.7,38.33 207.64,38.33 210.98,34.99 218.61,34.99 U1.58
SCL_S4_U  (via drill 0.5)
  Top 1.016: SCL.TP 66.6,52.33 68.23,50.85 68.23,42.72 69.91,41.12 94.35,41.05 98.95,36.41 98.93,30.2 v98.77,30.15 | v103.41,30.22 103.41,31.98 105.75,34.32 113.27,34.32 SCL_S4_C4_C2.TP
  Bottom 1.016: v98.77,30.15 103.34,30.15 v103.41,30.22
SCL_S4_U_1  (via drill 0.5)
  Top 1.016: R25.1 v4.77,31.04 4.77,32.77 SCL2.TP
  Bottom 0.305: U5.5 30.04,33.52 29.68,33.88 5.89,33.88 SCL2.TP 4.94,31.21 v4.77,31.04
SDA_S1  (via drill 0.6)
  Top 0.305: U1.3 218.79,27.76 217.32,26.27 v216.1,26.27 | R6.2 206.98,31.89 v207.54,32.49
  Bottom 0.305: 208.38,31.27 207.95,30.84 207.95,29.58 U2.4 | v216.1,26.27 216.1,30.08 214.91,31.27 208.38,31.27 | v207.54,32.49 207.72,32.51 207.86,32.31 207.84,31.8 208.38,31.27
SDA_S2
  Top 0.305: 218.71,39.13 U1.52 | SDA_S2_C1.TP 182.77,37.24 183.82,36.19 183.82,34.82 184.88,33.76 196.7,33.76 202.07,39.13
  Top 0.32: 202.07,39.13 218.71,39.13
SDA_S2_U  (via drill 0.6)
  Top 1.016: SDA_S2_C2_C2.TP 164.77,37.21 v160.41,32.89 159.69,33.56 159.69,44.23 R12.2
  Bottom 0.406: U3.4 149.41,31.03 150.54,32.17 159.66,32.17 v160.41,32.89
SDA_S3
  Top 0.305: SDA_S3_C1.TP 195.75,15.57 196.06,15.88 214.02,15.88 U1.13
SDA_S3_U  (via drill 0.5)
  Top 0.35: v92.06,31.32 92.06,24.92 93.34,23.64 98.31,23.64 v103.31,18.65
  Top 0.813: R26.1 87.98,12.07 89.14,13.23 105.19,13.23 v107.05,15.09 107.32,15.36 113.22,15.36 SDA_S3_C3_C4.TP
  Bottom 0.35: U4.4 88.24,30.54 89.14,31.44 91.94,31.44 v92.06,31.32 | v103.31,18.65 103.49,18.65 v107.05,15.09
SDA_S4
  Top 0.305: SDA_S4_C1.TP 182.57,31.83 182.94,32.2 200.55,32.2 201.83,33.48
  Top 0.32: 201.83,33.48 202.03,33.68 219.21,33.68 U1.59
SDA_S4_U  (via drill 0.5)
  Top 1.016: SDA.TP 65.4,49.3 66.77,47.99 66.77,41.41 69.03,39.14 92.6,39.14 97.06,34.68 97.06,29.63 v97.06,27.98 | v103.41,28.03 107.13,28.03 108.6,29.49 108.6,30.88 109.55,31.83 113.43,31.83 | 114.29,31.83 113.43,31.83 | 113.43,31.83 SDA_S4_C4_C4.TP
  Bottom 1.016: v97.06,27.98 v103.41,28.03
SDA_S4_U_1  (via drill 0.5)
  Top 1.016: R24.1 8.01,26.48 9.1,27.57 v9.1,32.55 9.1,35.11 8.55,35.67 4.88,35.67 SDA2.TP
  Bottom 0.305: U5.4 29.29,32.58 28.8,33.06 9.61,33.06 v9.1,32.55
SWDCLK  (via drill 0.6)
  Top 0.305: R2.2 200,50.91 v199.97,51.36 | 229,19.37 229,23.18 U1.21 | v226.24,18.32 227.95,18.32 229,19.37 | 229,19.37 229,19.34 228.73,19.07
  Bottom 0.305: v199.97,51.36 200.05,51.29 226.97,51.29 228.42,49.84 228.42,23.09 226.64,21.31 226.59,21.31 226.26,20.98 226.26,18.33 v226.24,18.32
SWDIO  (via drill 0.6)
  Top 0.305: R3.2 202.66,52.76 v202.76,52.86 | U1.20 228.37,23.11 228.37,20.37 227.88,19.89 v227.61,19.89
  Bottom 0.305: v202.76,52.86 227.68,52.86 229.66,50.88 229.69,21.87 v227.61,19.89
VCC_C2  (via drill 0.6)
  Top 2.184: 135.52,44.71 135.53,44.69 | 135.53,44.69 136.43,43.79 136.43,42.84 | VCC_C2_C3.TP 123.19,49.64 123.65,49.18 123.65,46.06 125.01,44.69 135.53,44.69
  Top 2.54: 170.78,47.53 v171.48,47.53 VCC_C2.TP | 136.43,42.84 v136.47,42.81 | v155.07,41.36 149.62,41.36 147.11,43.87
  Top 3.2: U$2.IN+ 149.46,54.06 147.11,51.71 147.11,43.87 147.11,42.22 145.11,40.21 138.34,40.21 136.47,42.09 v136.47,42.81
  Bottom 2.54: v171.48,47.53 171.43,47.47 171.43,42.53 170.94,42.04 170.94,41.87 169.53,40.46 162.34,40.46 161.61,39.73 VCC_2_C2.TP 156.67,39.76 v155.07,41.36 | v136.47,42.81 136.47,40.42 135.33,39.27
  Bottom 3.2: VCC_4_C2.TP 159.55,15.67 156.5,12.63 156.5,12.57 155.68,11.75 139.55,11.75 VCC_1_C2.TP 135.61,15.87 131.29,20.19 131.29,35.24 135.33,39.27 VCC_3_C2.TP
  pour Top (isolate 0.813): 120.89,0.4 174.15,0.36 174.33,10.3 172.91,10.36 173.34,45.68 174,45.55 174.09,55.49 120.84,55.46 121.09,46.03 122.21,45.99 122.56,9.88 120.72,9.77
VCC_C3  (via drill 0.6)
  Top 2.184: v111.71,45.89 111.71,49.57 | VCC.TP v101.33,49.5 v101.33,49.51
  Top 2.54: 111.71,49.57 VCC_C3.TP
  Bottom 2.184: v101.33,49.51 103.96,52.14 109.86,52.14 111.64,50.36 111.64,45.96 v111.71,45.89
  Bottom 3.2: v111.71,45.89 111.68,45.85 111.68,40.56 110.7,39.59 VCC_3_C3.TP 95.09,42.93 78.16,42.93 74.7,39.47 VCC_4_C3.TP 70.22,35.2 70.22,19.79 74.47,15.54 VCC_1_C3.TP 78.46,11.64 94.7,11.64 98.56,15.5 VCC_2_C3.TP
  pour Top (isolate 0.813): 58.95,0.21 112.27,0.2 112.04,10.41 114.55,10.3 114.77,45.03 112.82,45.05 112.58,55.08 58.69,55.24
VCC_C4  (via drill 0.6)
  Top 2.54: C2.+ 2.71,13.73 D1.C 2.82,16.33 3.44,16.95 14.67,16.95 v17.89,13.74 | VCC2.TP 37.26,52.96 42.32,47.91 42.32,37.39 v42.79,36.92 | BATTERY+.TP 33.95,7.05 32.91,8.08 32.91,11.7 v32.8,11.81
  Bottom 3.2: VCC_1_C4.TP v17.89,13.74 19.81,11.81 v32.8,11.81 35.32,11.81 39.64,16.13 VCC_2_C4.TP 42.79,19.46 v42.79,36.92 VCC_3_C4.TP | VCC_3_C4.TP | VCC_4_C4.TP 15.76,40.24 19.44,43.93 35.78,43.93 VCC_3_C4.TP
  pour Top (isolate 0.762): -0.02,0.75 55.02,0.37 55.05,55.2 0.1,55.26 -0.01,7.71
VCCC  (via drill 0.6)
  Top 2.184: C1.+ 225.62,12.98 v225.58,13.02
  Top 2.54: VCC_C1.TP 188.75,47.53 189.44,46.83 189.44,39.48 v191.64,37.28
  Bottom 1.676: DINA.2 226.82,4.03 227.54,4.75 228.19,4.75 228.93,5.49 228.93,11.03 226.98,12.98 225.62,12.98 v225.58,13.02
  Bottom 2.184: v225.58,13.02 225.58,13.21 223.16,15.62 218.09,15.62 VCC_1_C1.TP
  Bottom 3.2: VCC_1_C1.TP 216.68,15.77 213.48,12.57 196.96,12.57 VCC_2_C1.TP 190.46,19.08 190.46,36.1 v191.64,37.28 VCC_4_C1.TP 197.07,42.7 212.33,42.7 215.44,39.59 VCC_3_C1.TP
  pour Top (isolate 0.762): 180.28,54.99 180.39,44.88 178.34,45.06 178.51,10.52 180.09,10.49 180.31,0.14 233.17,0.03 233.17,55.02
VCCD
  Top 0.305: U1.48 226.08,36.53 225.4,37.21 225.4,39.74 C7.1
VDDA
  Top 0.305: 196.52,17.5 196.6,17.5 | 196.6,17.5 214.24,17.5 U1.11 221.67,24.95 221.72,24.95 223.13,26.37 223.13,31.88 U1.56 | VDDA_C1.TP 181.98,21.04 183.25,19.77 194.33,19.77 196.6,17.5
VDDA2  (via drill 0.6)
  Top 0.813: L1.2 161.14,8.39 163.52,8.39 164.34,9.2 164.34,12.36 166.35,14.37 v167.07,14.37 | v167.33,21.04 VDDA_C2.TP
  Bottom 0.813: v167.07,14.37 167.33,14.63 v167.33,21.04
VDDD  (via drill 0.6)
  Top 0.305: 181.28,53.14 VDDD_C1.TP 181.23,53.18 196.54,53.18 197.98,51.74 v197.98,45.09 | U1.50 220.95,38.32 218.1,41.17 218.1,44.29 v217.31,45.09
  Bottom 0.305: v217.31,45.09 v197.98,45.09
VDDD2
  Top 0.813: VDDD_C2.TP
  Top 1.27: L2.2 VDDD_C2.TP
VDDIO
  Top 0.27: 214.46,15.07 214.63,15.07 216.39,16.83 216.43,16.83 216.56,16.95 228.65,16.95 229.87,18.17 229.87,25.86 229.81,25.91
  Top 0.28: 186.33,14.66 196.15,14.66 196.56,15.07 214.46,15.07
  Top 0.305: U1.26 229.81,25.91 | VDDIO_C1.TP 179.47,13.01 184.68,13.01 186.33,14.66
VDDIO2
  Top 0.813: R15.2 165.31,5.43 165.92,6 165.88,11.84 167.08,12.93 171.17,12.93 VDDIO_C2.TP
XRES
  Top 0.305: U1.47 227.25,36.88 227.25,44.1 226.62,44.73 224,44.73 223.21,45.52 223.21,47.56 R14.2 C10.1 223.22,49.58 R1.2

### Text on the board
bNames: EMERGE FACE 4 | EMERGE FACE 3 | EMERGE FACE 2 | EMERGE FACE 1

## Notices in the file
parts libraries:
diy-modules: Released under the Creative Commons Attribution 4.0 International License: http://creativecommons.org/licenses/by/4.0
